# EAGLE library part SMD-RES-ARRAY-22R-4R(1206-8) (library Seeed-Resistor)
301030014
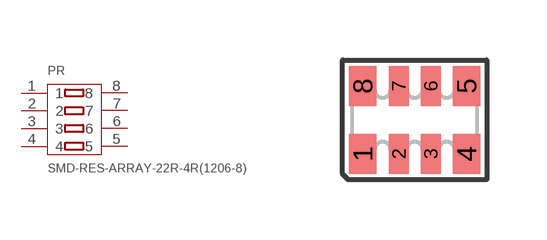
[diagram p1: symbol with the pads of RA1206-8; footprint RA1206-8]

Designator prefix PR

## SMD-RES-ARRAY-22R-4R(1206-8) (MPN: YC324-JK-0722RL; VALUE: 22R-4R)  [RA1206-8]
1  1
2  2
3  3
4  4
5  5
6  6
7  7
8  8

## Footprint RA1206-8 (pad centres in mm)
BOURNS Chip Resistor Array Source: RS Component / BUORNS
smd 0.7 x 1: 1 -1.3,-0.85; 4 1.3,-0.85; 5 1.3,0.85; 8 -1.3,0.85
smd 0.5 x 1: 2 -0.4,-0.85; 3 0.4,-0.85; 6 0.4,0.85; 7 -0.4,0.85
